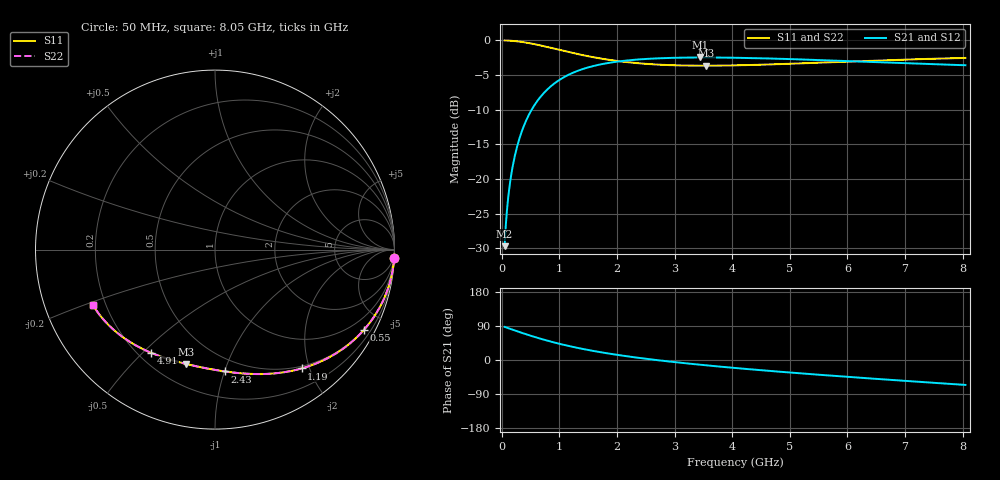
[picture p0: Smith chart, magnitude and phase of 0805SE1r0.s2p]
! AVX Thin Film Operation		Date: August 2001
! Description: Accu-P® Series, Thin Film, SMD, RF Capacitor
! Part Number: 08051J1R0ABT
! 50 MHz  -  8.05 GHz
! Serial Measurements
# mhz S db R 50
!	S11		S21		S12		S22
!	dB	Phase	dB	Phase	dB	Phase	dB	Phase
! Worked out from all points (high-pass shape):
!   401 points, 50 MHz to 8.05 GHz, reference 50 ohm
!   highest |S21| = -2.46 dB at 3.45 GHz (marker M1); lowest = -29.7 dB at 50 MHz (marker M2)
!   |S21| within 3 dB of the highest: 1.048 GHz to end of sweep
!   lowest |S11| = -3.6 dB at 3.55 GHz (marker M3), VSWR 4.83, Z = 16.2 - j36.4 ohm
!   |S11| at or under -10 dB: nowhere
!   |S22| runs from -3.6 to 0.0 dB; largest |S21 - S12| = 8.4e-05
!   S11 on the Smith chart (normalised r, x): 50 MHz: 0, -43; 550 MHz: 0.49, -3.93; 1.19 GHz: 0.47, -1.88; 2.43 GHz: 0.40, -1.00; 4.91 GHz: 0.25, -0.53; 8.05 GHz: 0.15, -0.21
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50  -0.00 -2.7  -29.69 87.3  -29.69 87.3  -0.00 -2.7
70  -0.01 -3.7  -26.78 86.3  -26.78 86.3  -0.01 -3.7
110  -0.02 -5.9  -22.87 84.1  -22.87 84.1  -0.02 -5.9
150  -0.04 -8.0  -20.20 82.0  -20.20 82.0  -0.04 -8.0
230  -0.10 -12.2  -16.57 77.8  -16.57 77.8  -0.10 -12.2
290  -0.15 -15.3  -14.63 74.7  -14.63 74.7  -0.15 -15.3
370  -0.24 -19.4  -12.64 70.6  -12.64 70.6  -0.24 -19.4
550  -0.51 -28.2  -9.58 61.8  -9.58 61.8  -0.51 -28.2
690  -0.76 -34.5  -7.98 55.4  -7.98 55.4  -0.76 -34.5
850  -1.06 -41.3  -6.64 48.7  -6.64 48.7  -1.06 -41.3
1190  -1.73 -53.9  -4.84 36.1  -4.84 36.1  -1.73 -53.9
1390  -2.10 -60.3  -4.18 29.7  -4.18 29.7  -2.10 -60.3
1870  -2.81 -73.2  -3.23 16.7  -3.23 16.7  -2.81 -73.2
2430  -3.33 -85.3  -2.71 4.6  -2.71 4.6  -3.33 -85.3
2730  -3.50 -90.9  -2.58 -0.9  -2.58 -0.9  -3.50 -90.9
3450  -3.65 -102.5  -2.46 -12.6  -2.46 -12.6  -3.65 -102.5
3550  -3.65 -104.0  -2.46 -14.1  -2.46 -14.1  -3.65 -104.0
4050  -3.60 -111.0  -2.50 -21.1  -2.50 -21.1  -3.60 -111.0
4910  -3.40 -121.9  -2.67 -31.9  -2.67 -31.9  -3.40 -121.9
5390  -3.25 -127.5  -2.80 -37.6  -2.80 -37.6  -3.25 -127.5
6730  -2.84 -142.1  -3.21 -52.2  -3.21 -52.2  -2.84 -142.1
8050  -2.53 -155.7  -3.58 -65.8  -3.58 -65.8  -2.53 -155.7
